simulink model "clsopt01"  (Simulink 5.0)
settings: Solver=ode45  SolverMode=SingleTasking  StartTime=0.0  StopTime=100  FixedStep=1  MaxStep=1  RelTol=1e-3  AbsTol=1e-6
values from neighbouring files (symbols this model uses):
  D = par(3)    [trackfun.m]
  I = par(2)    [trackfun.m]
  P = par(1)    [trackfun.m]    (also in demo_rarxcup.m = 1.0*eye(2); demo_rarxup.m = 1.0*eye(2); drec1.m = 1.e5*eye(d); rarxcup.m = W - Q)

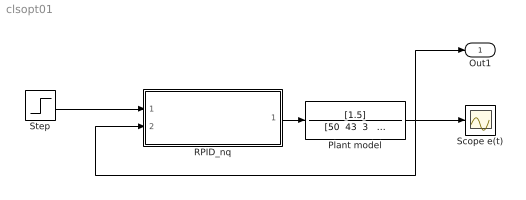
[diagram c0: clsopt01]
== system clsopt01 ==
  Plant model : TransferFcn  Numerator=[1.5]  Denominator="[50  43  3   1]"
  RPID_nq : Subsystem  mask( PID ){P=P, I=I, D=D, h=1}
      mask prompts: P "P :"; I "I [s]:"; D "D [s]:"; h "h [s]:"
      mask help: PID : P, I, D - ; h - ;
      mask init:
      | %  Documentation
      |                 P=@1;  I=@2;  D=@3;  h=@4;
      | q2=P*(D/h);  q0=P+q2;  q1=-P+P*(h/I)-2*q2;
  Scope e(t) : Scope
  Step : Step  Time=0  SampleTime=1
  Out1 : Outport
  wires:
  Plant model/1 -> Scope e(t)/1, RPID_nq/2(In2), Out1/1
  RPID_nq/1(Out1) -> Plant model/1
  Step/1 -> RPID_nq/1(In1)

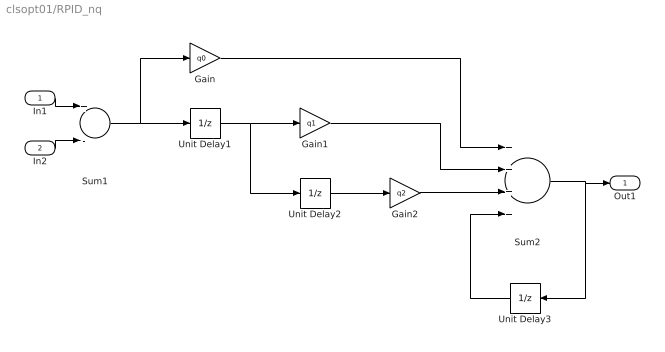
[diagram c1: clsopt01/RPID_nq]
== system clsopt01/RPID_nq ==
  In1 : Inport
  In2 : Inport  Port=2
  Gain : Gain  Description=GAIN 0  Gain=q0
  Gain1 : Gain  Description=Gain 1  Gain=q1
  Gain2 : Gain  Gain=q2
  Sum1 : Sum  Inputs=+-
  Sum2 : Sum  Inputs=++++
  Unit Delay1 : UnitDelay  Description=Gain 0
  Unit Delay2 : UnitDelay  Description=Gain 1
  Unit Delay3 : UnitDelay  Orientation=left
  Out1 : Outport  InitialOutput=0
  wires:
  Sum1/1 -> Unit Delay1/1, Gain/1
  Gain/1 -> Sum2/1
  Unit Delay1/1 -> Gain1/1, Unit Delay2/1
  Unit Delay2/1 -> Gain2/1
  Gain1/1 -> Sum2/2
  Gain2/1 -> Sum2/3
  Sum2/1 -> Unit Delay3/1, Out1/1
  Unit Delay3/1 -> Sum2/4
  In1/1 -> Sum1/1
  In2/1 -> Sum1/2
